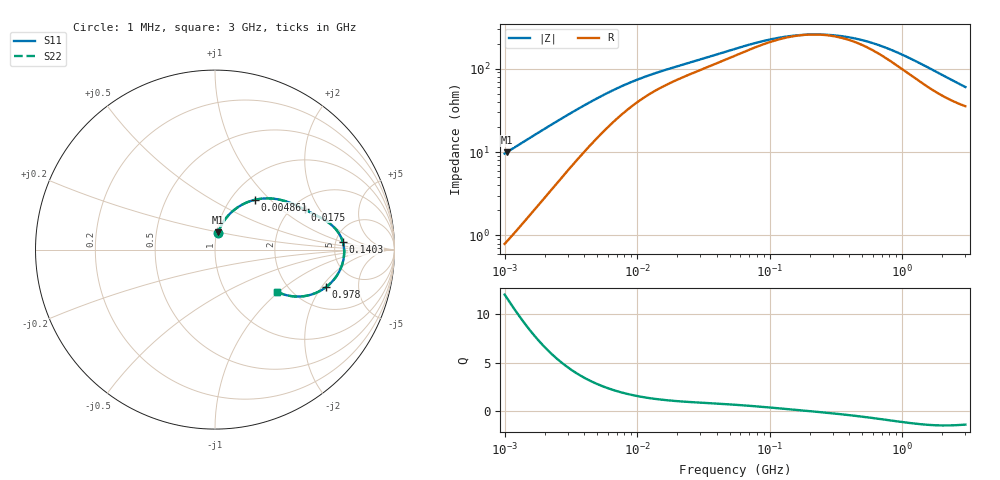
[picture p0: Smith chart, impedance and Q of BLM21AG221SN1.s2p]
! BLM21AG221SN1
# Hz S RI R 50
!Freq.(Hz) S11(Real) S11(Imag) S21(Real) S21(Imag) S12(Real) S12(Imag) S22(Real) S22(Imag)
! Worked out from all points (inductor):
!   401 points, 1 MHz to 3 GHz, reference 50 ohm
!   read as one part in series: L = 1.51 uH near 1.041 MHz
!   highest Q = 11.7 at 1.041 MHz (marker M1), where L = 1.52 uH
!   self-resonance near 206.1 MHz
!   S11 on the Smith chart (normalised r, x): 1 MHz: 1.02, +0.19; 4.861 MHz: 1.28, +0.81; 17.5 MHz: 2.33, +1.49; 140.3 MHz: 5.79, +1.01; 978 MHz: 3.02, -2.21; 3 GHz: 1.71, -0.97
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1000000  0.0167 0.0932  0.9833 -0.0932  0.9833 -0.0932  0.0167 0.0932
1040844  0.018 0.0968  0.982 -0.0968  0.982 -0.0968  0.018 0.0968
2139570  0.0661 0.1809  0.9339 -0.1809  0.9339 -0.1809  0.0661 0.1809
2888807  0.1088 0.2227  0.8912 -0.2227  0.8912 -0.2227  0.1088 0.2227
3823119  0.1646 0.2572  0.8354 -0.2572  0.8354 -0.2572  0.1646 0.2572
4861065  0.2228 0.2775  0.7772 -0.2775  0.7772 -0.2775  0.2228 0.2775
8017732  0.3519 0.2798  0.6481 -0.2798  0.6481 -0.2798  0.3519 0.2798
1.461624e7  0.472 0.2372  0.528 -0.2372  0.528 -0.2372  0.472 0.2372
1.750132e7  0.4996 0.2235  0.5004 -0.2235  0.5004 -0.2235  0.4996 0.2235
5.477226e7  0.6448 0.1412  0.3552 -0.1412  0.3552 -0.1412  0.6448 0.1412
9.402997e7  0.6924 0.0869  0.3076 -0.0869  0.3076 -0.0869  0.6924 0.0869
1.403209e8  0.7119 0.0429  0.2881 -0.0429  0.2881 -0.0429  0.7119 0.0429
2.094008e8  0.7195 -0.00179  0.2805 0.00179  0.2805 0.00179  0.7195 -0.00179
2.942768e8  0.718 -0.0413  0.282 0.0413  0.282 0.0413  0.718 -0.0413
4.0536e8  0.709 -0.0818  0.291 0.0818  0.291 0.0818  0.709 -0.0818
5.583748e8  0.6899 -0.1267  0.3101 0.1267  0.3101 0.1267  0.6899 -0.1267
8.005644e8  0.6504 -0.1808  0.3496 0.1808  0.3496 0.1808  0.6504 -0.1808
9.779672e8  0.6177 -0.2098  0.3823 0.2098  0.3823 0.2098  0.6177 -0.2098
1.320433e9  0.5536 -0.2449  0.4464 0.2449  0.4464 0.2449  0.5536 -0.2449
1.712864e9  0.4869 -0.2604  0.5131 0.2604  0.5131 0.2604  0.4869 -0.2604
2.221924e9  0.4177 -0.258  0.5823 0.258  0.5823 0.258  0.4177 -0.258
3e9  0.3461 -0.2349  0.6539 0.2349  0.6539 0.2349  0.3461 -0.2349
